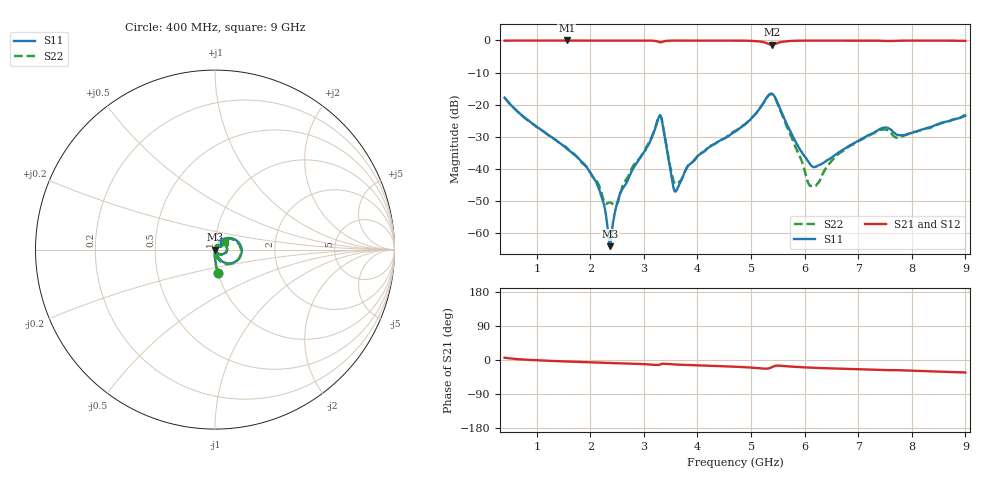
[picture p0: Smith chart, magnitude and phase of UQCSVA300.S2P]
!  Part Number  UQCSVA300  Mounting Orientation: Horizontal
!  Description: Ultra Low ESR Microwave capacitors
!  Application: Coupling, Bypass, Tuning, DC Block
!  Filters, Matching
# GHZ S DB R 50
! Freq  |S11|  S11 Ph  |S21|  S21 Ph  |S12|  S12 Ph  |S22|  S22 Ph
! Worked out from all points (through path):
!   801 points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, 400 MHz to 9 GHz, reference 50 ohm
!   highest |S21| = -0.01 dB at 1.561 GHz (marker M1); lowest = -1.4 dB at 5.388 GHz (marker M2)
!   group delay of S21, straight-line fit = 10.7 ps
!   lowest |S11| = -64.1 dB at 2.367 GHz (marker M3), VSWR 1.00, Z = 49.9 + j0.0149 ohm
!   |S11| at or under -10 dB: start of sweep to end of sweep
!   |S22| runs from -51.5 to -16.7 dB; largest |S21 - S12| = 0.0026
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0.4  -17.81 -83.3  -0.08 6.1  -0.09 6.1  -17.81 -83.5
1.561  -33.70 -94.4  -0.01 -3.9  -0.02 -4.0  -33.39 -91.2
1.841  -37.80 -95.8  -0.01 -5.3  -0.02 -5.3  -38.08 -90.2
2.142  -45.36 -104.3  -0.01 -6.8  -0.02 -6.8  -44.45 -77.0
2.271  -52.36 -101.8  -0.01 -7.3  -0.02 -7.3  -50.62 -58.8
2.367  -64.06 166.2  -0.02 -7.8  -0.03 -7.8  -50.43 -19.9
2.475  -52.30 77.7  -0.02 -8.3  -0.03 -8.3  -51.41 21.6
2.561  -47.43 81.2  -0.02 -8.6  -0.03 -8.6  -47.54 44.9
3.088  -32.41 70.1  -0.05 -11.6  -0.06 -11.6  -32.05 63.0
3.27  -24.25 30.9  -0.42 -13.1  -0.43 -13.2  -24.02 25.7
3.346  -25.89 -29.7  -0.43 -9.9  -0.44 -10.0  -25.57 -33.4
3.507  -41.51 -46.4  -0.07 -11.3  -0.08 -11.3  -40.59 -46.6
3.593  -47.07 9.5  -0.05 -12.0  -0.06 -12.0  -44.65 0.9
4.001  -36.04 68.3  -0.02 -14.2  -0.04 -14.2  -35.99 64.7
4.7  -28.42 62.8  -0.06 -17.7  -0.07 -17.7  -28.23 62.9
5.388  -16.56 -9.5  -1.36 -19.0  -1.37 -19.0  -16.74 -13.5
6.065  -37.67 -36.1  -0.06 -19.9  -0.07 -19.9  -44.37 -50.1
6.141  -39.19 -22.4  -0.05 -20.4  -0.07 -20.4  -45.16 -18.7
6.624  -34.97 35.5  -0.04 -22.8  -0.06 -22.8  -35.38 56.3
7.57  -27.37 28.2  -0.18 -26.7  -0.20 -26.7  -28.19 28.7
7.871  -29.43 38.4  -0.07 -27.5  -0.09 -27.4  -29.59 43.6
9  -23.44 48.2  -0.14 -33.0  -0.16 -32.9  -23.17 39.5
